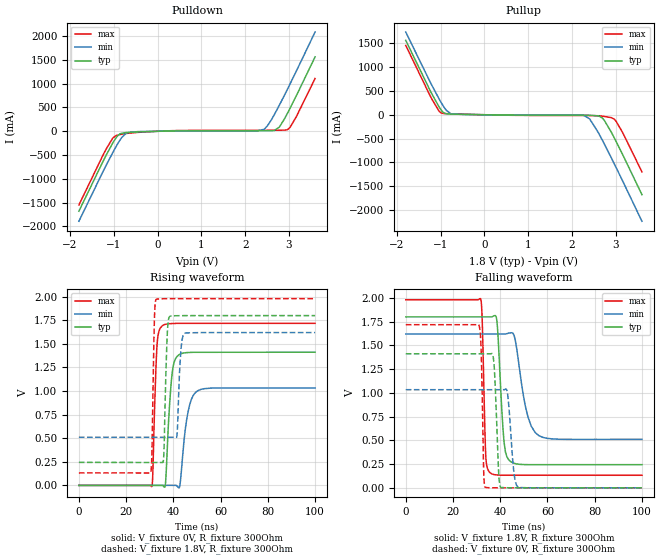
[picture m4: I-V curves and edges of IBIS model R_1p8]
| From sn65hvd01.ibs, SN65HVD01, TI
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|   Model
[Model]   R_1p8
Model_type   Output
Polarity   Non-Inverting
Vmeas = 0.9
Vref = 0
Cref = 1pF
Rref = 100000
|   typ   min   max
C_comp   1.990pF   1.630pF   2.168pF
[Voltage Range]   1.8   1.62   1.98
[Temperature Range]   27   125   -40
[Pullup Reference]   1.8   1.62   1.98
[Pulldown Reference]   -0   -0   -0
[Power Clamp Reference]   1.8   1.62   1.98
[GND Clamp Reference]   -0   -0   -0
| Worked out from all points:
|   slope of the pulldown table from 0 to 0.27 V, typ, clamps not added: 48.4 ohm
|   slope of the pullup table from 0 to 0.27 V, typ, clamps not added: 76.6 ohm
|   falling waveform, V_fixture 1.8V, R_fixture 300Ohm: 20-80 % time 2.07ns typ, 4.59ns min, 1.08ns max; typ from 1.8 V to 0.244 V
|   rising waveform, V_fixture 0V, R_fixture 300Ohm: 20-80 % time 2.01ns typ, 3.08ns min, 1.31ns max; typ from 0 V to 1.41 V
|   rising waveform, V_fixture 1.8V, R_fixture 300Ohm: 20-80 % time 1.01ns typ, 1.18ns min, 786ps max; typ from 0.244 V to 1.8 V
|   falling waveform, V_fixture 0V, R_fixture 300Ohm: 20-80 % time 1.34ns typ, 1.84ns min, 845ps max; typ from 1.41 V to 0 V
[Pulldown]
|   Voltage   I(typ)   I(min)   I(max)
-1.795V   -1.68A     -1.891A    -1.55A
-1.255V   -652.8mA   -866.7mA   -520.8mA
-1.022V   -247mA     -449.6mA   -143.8mA
-855mV    -53.79mA   -181.9mA   -68.55mA
-703.8mV  -25.14mA   -31.69mA   -44.55mA
2.261V    10.99mA    5.637mA    20.82mA
2.439V    11.37mA    45.81mA    20.99mA
2.666V    16.6mA     351.3mA    21.74mA
2.779V    88.76mA    547.2mA    22.62mA
2.995V    432mA      941.6mA    54.58mA
3.168V    748.5mA    1.267A     309.2mA
3.595V    1.563A     2.086A     1.109A
[Pullup]
|   Voltage   I(typ)   I(min)   I(max)
-1.795V   1.563A     1.738A     1.457A
-1.255V   539.4mA    719.4mA    428.5mA
-1.033V   162.7mA    331mA      72.98mA
-903.6mV  29.11mA    135.9mA    24.47mA
-763.2mV  13.63mA    20.06mA    20.37mA
2.207V    -9.102mA   -6.241mA   -16.51mA
2.401V    -10.48mA   -86.84mA   -16.82mA
2.612V    -27.87mA   -396.3mA   -22.56mA
2.693V    -70.98mA   -536.6mA   -30.33mA
2.974V    -504mA     -1.05A     -102.6mA
3.157V    -842.5mA   -1.397A    -379.3mA
3.595V    -1.68A     -2.239A    -1.2A
[Ramp]
R_load = 300
|   typ   min   max
dV/dt_r   0.847062/2.00836e-09   0.619974/3.07747e-09   1.03068/1.30627e-09
dV/dt_f   0.933637/2.07495e-09   0.665731/4.58892e-09   1.10855/1.08088e-09
[Falling Waveform]
V_fixture = 1.8V
V_fixture_min = 1.62V
V_fixture_max = 1.98V
R_fixture = 300Ohm
C_fixture = 0F
|   Time   V(typ)   V(min)   V(max)
0s        1.8V       1.62V      1.98V
31.78ns   1.8V       1.62V      1.987V
32.48ns   1.8V       1.62V      1.674V
33.91ns   1.8V       1.62V      319.3mV
35.81ns   1.8V       1.62V      156.5mV
38.55ns   1.767V     1.62V      135.5mV
41.59ns   486.7mV    1.62V      132.6mV
44.02ns   284.2mV    1.631V     132.6mV
56.43ns   243.7mV    548.6mV    132.6mV
100ns     243.9mV    510.4mV    132.4mV
[Rising Waveform]
V_fixture = 0V
V_fixture_min = 0V
V_fixture_max = 0V
R_fixture = 300Ohm
C_fixture = 0F
|   Time   V(typ)   V(min)   V(max)
0s        1.126nV    39.3nV     543.6pV
30.89ns   241.7uV    320.3uV    -10.81mV
33.02ns   258.4uV    342.3uV    1.458V
35.28ns   276.1uV    365.7uV    1.691V
36.64ns   13.35mV    379.9uV    1.707V
39.53ns   1.196V     409.8uV    1.716V
42.2ns    1.382V     -24.65mV   1.718V
45.93ns   1.408V     739.6mV    1.718V
49.78ns   1.411V     993.7mV    1.718V
100ns     1.412V     1.033V     1.718V
[Rising Waveform]
V_fixture = 1.8V
V_fixture_min = 1.62V
V_fixture_max = 1.98V
R_fixture = 300Ohm
C_fixture = 0F
|   Time   V(typ)   V(min)   V(max)
0s        243.9mV    510.4mV    132.4mV
30.4ns    243.1mV    510.5mV    135.2mV
31.94ns   243.1mV    510.5mV    1.731V
32.69ns   243.1mV    510.5mV    1.971V
35.84ns   279.4mV    510.5mV    1.979V
37.44ns   1.614V     510.5mV    1.979V
38.55ns   1.793V     510.5mV    1.98V
41.52ns   1.799V     529.8mV    1.98V
44.53ns   1.8V       1.607V     1.98V
100ns     1.8V       1.62V      1.98V
[Falling Waveform]
|Gnd
V_fixture = 0V
V_fixture_min = 0V
V_fixture_max = 0V
R_fixture = 300Ohm
C_fixture = 0F
|   Time   V(typ)   V(min)   V(max)
0s        1.412V     1.033V     1.718V
31ns      1.412V     1.033V     1.713V
31.78ns   1.412V     1.033V     1.541V
33.02ns   1.412V     1.033V     159.3mV
33.72ns   1.412V     1.033V     4.522mV
37.13ns   1.361V     1.033V     542.6uV
40.18ns   4.701mV    1.033V     174.6uV
43.03ns   992.8uV    1.002V     166.2uV
47.67ns   245.2uV    6.401mV    152.7uV
100ns     -259.7nV   2.137uV    -17.57nV
